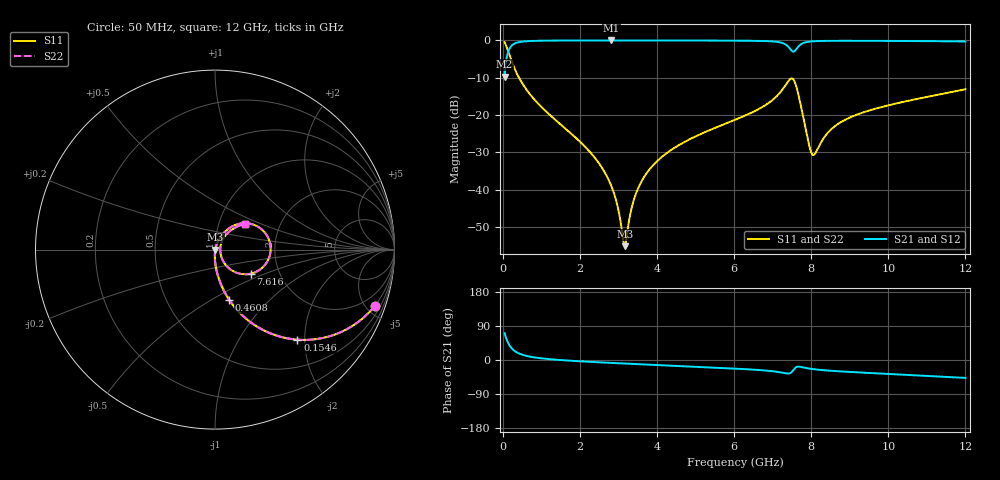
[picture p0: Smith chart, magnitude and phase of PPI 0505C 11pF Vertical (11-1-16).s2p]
# GHz S MA R 50
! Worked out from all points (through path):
!   1601 points, 50 MHz to 12 GHz, reference 50 ohm
!   highest |S21| = -0.02 dB at 2.821 GHz (marker M1); lowest = -9.7 dB at 50 MHz (marker M2)
!   group delay of S21, straight-line fit = 13.4 ps
!   lowest |S11| = -55.1 dB at 3.164 GHz (marker M3), VSWR 1.00, Z = 50.2 - j0.0273 ohm
!   |S11| at or under -10 dB: 424.2 MHz to end of sweep
!   |S22| runs from -55.1 to -0.5 dB; largest |S21 - S12| = 0
!   S11 on the Smith chart (normalised r, x): 50 MHz: 0.99, -5.71; 154.6 MHz: 0.99, -1.84; 460.8 MHz: 0.99, -0.61; 7.616 GHz: 1.43, -0.41; 12 GHz: 1.33, +0.41
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0.05  0.9446 -19.3  0.3282 70.7  0.3282 70.7  0.9446 -19.3
0.1545625  0.6805 -47.5  0.7324 42.4  0.7324 42.4  0.6805 -47.5
0.2740625  0.4622 -63.2  0.8862 26.7  0.8862 26.7  0.4622 -63.2
0.4607812  0.2925 -74.2  0.9555 15.6  0.9555 15.6  0.2925 -74.2
0.9985312  0.1294 -85.1  0.9905 4.5  0.9905 4.5  0.1294 -85.1
2.044156  0.04204 -91.7  0.9976 -3.7  0.9976 -3.7  0.04204 -91.7
2.514687  0.02196 -92.1  0.998 -6.2  0.998 -6.2  0.02196 -92.1
2.820906  0.01112 -89.2  0.9981 -7.7  0.9981 -7.7  0.01112 -89.2
2.962813  0.006542 -83.4  0.9981 -8.4  0.9981 -8.4  0.006542 -83.4
3.164469  0.001757 -8.9  0.998 -9.4  0.998 -9.4  0.001757 -8.9
3.493094  0.009928 68.3  0.9979 -10.9  0.9979 -10.9  0.009928 68.3
4.038312  0.02507 72.0  0.9974 -13.4  0.9974 -13.4  0.02507 72.0
6.025  0.08646 64.7  0.9919 -22.7  0.9919 -22.7  0.08646 64.7
6.854031  0.1403 56.9  0.9776 -28.1  0.9776 -28.1  0.1403 56.9
7.309625  0.2403 37.1  0.8977 -34.6  0.8977 -34.6  0.2403 37.1
7.488875  0.3099 3.5  0.7319 -32.4  0.7319 -32.4  0.3099 3.5
7.615844  0.2403 -33.9  0.7658 -18.6  0.7658 -18.6  0.2403 -33.9
7.772687  0.1071 -55.0  0.9108 -19.1  0.9108 -19.1  0.1071 -55.0
8.019156  0.03023 -14.1  0.9697 -23.7  0.9697 -23.7  0.03023 -14.1
8.743625  0.07891 53.7  0.9876 -30.0  0.9876 -30.0  0.07891 53.7
10.01331  0.1355 50.9  0.9846 -36.8  0.9846 -36.8  0.1355 50.9
12  0.2217 40.8  0.9669 -47.3  0.9669 -47.3  0.2217 40.8
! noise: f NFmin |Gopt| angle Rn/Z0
0.05  0.0004005  0.8729  1.737  0.0006795
1.372  0.004052  0.6786  4.446  0.002434
2.701  0.006721  0.6301  8.094  0.003394
4.031  0.009276  0.607  11.72  0.004324
5.36  0.01253  0.6132  15.34  0.005915
6.682  0.02387  0.73  19.23  0.01713
8.012  0.04951  0.8353  23.38  0.06095
9.341  0.02443  0.6523  26.55  0.01269
10.67  0.02452  0.6163  29.7  0.01115
12  0.03022  0.6466  33.2  0.01495
